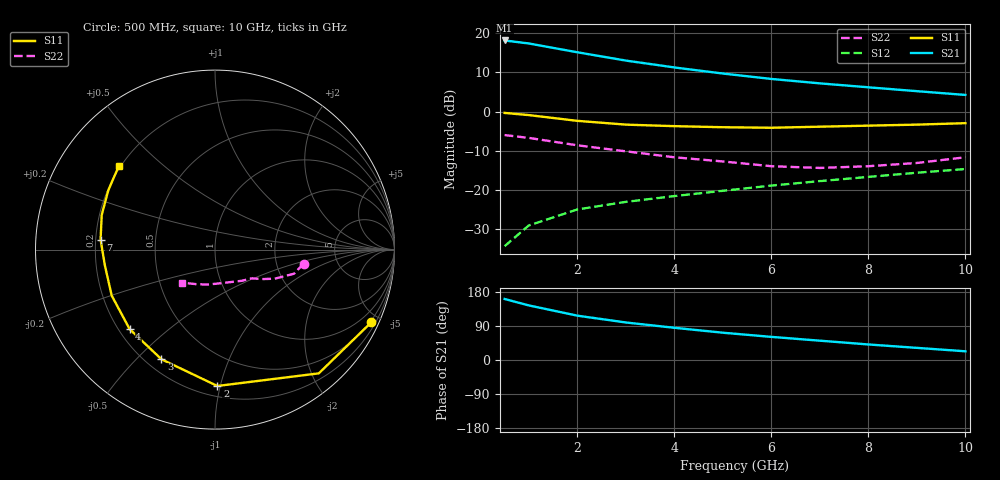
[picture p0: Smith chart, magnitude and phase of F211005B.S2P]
!ATF-21100
!S-PARAMETERS at Vds=5V  Id=80mA.  LAST UPDATED 07-22-92
# ghz s ma r 50
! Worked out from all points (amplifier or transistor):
!   11 points, 500 MHz to 10 GHz, reference 50 ohm
!   highest |S21| = 18.2 dB at 500 MHz (marker M1)
!   |S21| within 3 dB of that: start of sweep to 1.99 GHz
!   unconditionally stable (mu >= 1): 5.474 GHz to 6.96 GHz
!   at 1 GHz: K = 0.33, MSG = 23.3 dB, |S12| = -29.1 dB
!   at 5 GHz: K = 0.98, MSG = 15.0 dB, |S12| = -20.3 dB
!   at 10 GHz: K = 0.87, MSG = 9.5 dB, |S12| = -14.7 dB
!   S11 on the Smith chart (normalised r, x): 500 MHz: 0.43, -4.47; 2 GHz: 0.27, -0.98; 3 GHz: 0.26, -0.59; 4 GHz: 0.24, -0.37; 7 GHz: 0.22, +0.04; 10 GHz: 0.19, +0.36
0.5  0.96 -25.0  8.1 161.0  0.019 80.0  0.5 -9.0
1  0.9 -50.0  7.41 144.0  0.035 71.0  0.46 -17.0
2  0.76 -89.0  5.72 117.0  0.056 62.0  0.37 -26.0
3  0.68 -116.0  4.48 99.0  0.07 60.0  0.31 -32.0
4  0.65 -137.0  3.66 85.0  0.083 61.0  0.26 -38.0
5  0.63 -156.0  3.06 72.0  0.097 61.0  0.23 -49.0
6  0.62 -172.0  2.61 61.0  0.113 62.0  0.2 -65.0
7  0.64 175.0  2.29 51.0  0.129 61.0  0.19 -86.0
8  0.66 163.0  2.04 41.0  0.146 60.0  0.2 -103.0
9  0.68 151.0  1.82 32.0  0.165 57.0  0.22 -119.0
10  0.71 139.0  1.63 23.0  0.184 54.0  0.26 -135.0
